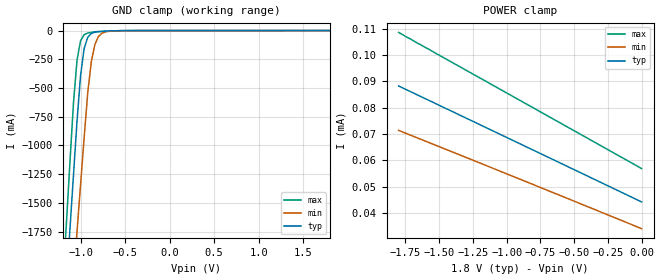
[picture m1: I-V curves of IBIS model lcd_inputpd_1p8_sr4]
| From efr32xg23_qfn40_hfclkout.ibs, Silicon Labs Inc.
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|   Model lcd_inputpd_1p8_sr4
[Model]  lcd_inputpd_1p8_sr4
Model_type Input
C_comp   1.6300pF   1.4000pF   2.7000pF
[Temperature Range]   25.0000   0.1250k   -40.0000
[Pullup Reference]   1.8000V   1.6200V   1.9800V
[Pulldown Reference]   0.0V   0.0V   0.0V
[POWER Clamp Reference]   1.8000V   1.6200V   1.9800V
[GND Clamp Reference]   0.0V   0.0V   0.0V
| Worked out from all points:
|   GND clamp passes 1 mA (typ) near -0.56 V on its own axis
[GND_clamp]
|Voltage   I(typ)   I(min)   I(max)
-1.8V     -9.867A    -9.569A    -10.32A
-1.2V     -2.688A    -3.389A    -2.224A
-1.16V    -2.211A    -2.978A    -1.687A
-1.12V    -1.735A    -2.567A    -1.152A
-1.08V    -1.26A     -2.157A    -630.4mA
-1.04V    -786.2mA   -1.747A    -256.2mA
-1V       -388.1mA   -1.338A    -87.59mA
-960mV    -155.8mA   -930mA     -35.75mA
-880mV    -25.04mA   -272.7mA   -16.3mA
-840mV    -13.93mA   -121.5mA   -10.47mA
-760mV    -7.83mA    -22.79mA   -6.546mA
1.8V      44.27uA    37.89uA    51.77uA
[POWER_clamp]
|Voltage   I(typ)   I(min)   I(max)
-1.8V     88.26uA    71.42uA    108.6uA
-1.66V    84.85uA    68.54uA    104.5uA
-880mV    65.81uA    52.45uA    82.19uA
0V        44.27uA    34.13uA    56.93uA
